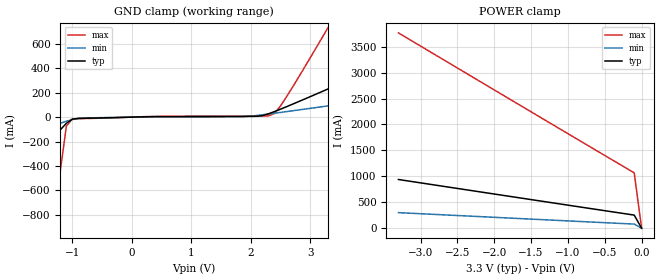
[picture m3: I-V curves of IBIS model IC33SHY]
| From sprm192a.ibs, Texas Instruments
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[Model]   IC33SHY
Model_type   Input
Polarity   Non-Inverting
| signals   A, Y
Vinl = 0.8V
Vinh = 2.0V
|   typ   min   max
C_comp   1.561p   1.515p   1.648p
|   typ   min   max
[Temperature Range]   25   -40   125
|   typ   min   max
[Voltage Range]   3.30V   3.00V   3.60V
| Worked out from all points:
|   POWER clamp passes 1 mA (typ) near -0.00 V on its own axis
[GND_clamp]
|   Voltage   I(typ)   I(min)   I(max)
-3.3V     -1.477A    -434.4mA   -12.61A
-2.5V     -943mA     -285mA     -7.87A
-1.4V     -223.8mA   -84.05mA   -1.479A
-1.3V     -162mA     -66.73mA   -935.5mA
-1.2V     -103mA     -49.93mA   -432mA
-1.1V     -50.35mA   -34.1mA    -73.5mA
-1V       -16.76mA   -20.26mA   -14.72mA
2.1V      6.87mA     13.4mA     8.831mA
2.3V      27.22mA    25.46mA    10.12mA
2.4V      45.36mA    31.84mA    29.43mA
2.5V      64.77mA    38.34mA    90.24mA
3.3V      230.7mA    92.11mA    732.9mA
[POWER_clamp]
|   Voltage   I(typ)   I(min)   I(max)
-3.3V     938.4mA    299.4mA    3.765A
-1.4V     529.6mA    167.7mA    2.16A
-100mV    251.9mA    78.51mA    1.067A
0V        1pA        1pA        1pA
